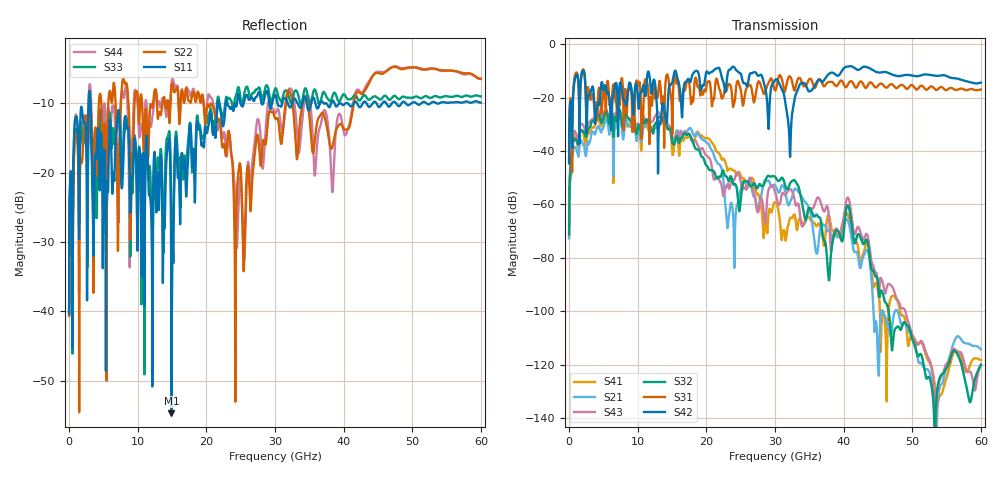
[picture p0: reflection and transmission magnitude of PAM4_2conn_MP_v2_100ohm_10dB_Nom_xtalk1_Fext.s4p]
! Info: Touchstone file created by Circ.  Input file=FAB50GbE_2conn_Midplane_Examax_Topo2_v2_100ohm_10dB_Nom.circ
# Hz S RI R 50
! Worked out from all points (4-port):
!   6000 points, 10 MHz to 60 GHz, reference 50 ohm
!   strongest paths, dB at 10 MHz, 15.01 GHz, 30.01 GHz, 45.01 GHz, 60 GHz:
!     S42: -44.6, -14.5, -13.5, -10.6, -14.4
!     S31: -44.0, -29.7, -17.3, -15.5, -17.0
!     S32: -71.3, -36.1, -49.7, -89.4, -120.0
!     S43: -71.5, -35.5, -55.2, -90.1, -120.1
!     S21: -72.7, -35.1, -52.9, -119.9, -114.3
!     S41: -67.7, -39.7, -59.3, -92.3, -118.3
!   lowest |S11| = -54.7 dB at 14.91 GHz (marker M1), VSWR 1.00, Z = 49.8 - j0.0612 ohm
!   |S11| at or under -10 dB: start of sweep to 2.839 GHz; 3.128 GHz to 21.66 GHz (18.53 GHz wide, 150 % of centre); 23.07 GHz to 24.47 GHz (1.397 GHz wide, 5.88 % of centre)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
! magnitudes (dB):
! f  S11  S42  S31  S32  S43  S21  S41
! 10 MHz  -40.3  -44.6  -44.0  -71.3  -71.5  -72.7  -67.7
! 4.14 GHz  -14.2  -23.0  -24.4  -26.8  -24.9  -31.2  -28.1
! 14.91 GHz  -54.7  -15.0  -20.7  -34.1  -34.4  -33.9  -36.1
! 24.07 GHz  -10.5  -8.7  -22.0  -52.4  -50.9  -83.8  -47.3
! 32.14 GHz  -10.6  -38.1  -12.0  -52.4  -54.3  -59.5  -65.6
! 37.84 GHz  -10.6  -11.2  -14.2  -88.2  -64.0  -69.8  -64.1
! 60 GHz  -9.9  -14.4  -17.0  -120.0  -120.1  -114.3  -118.3
